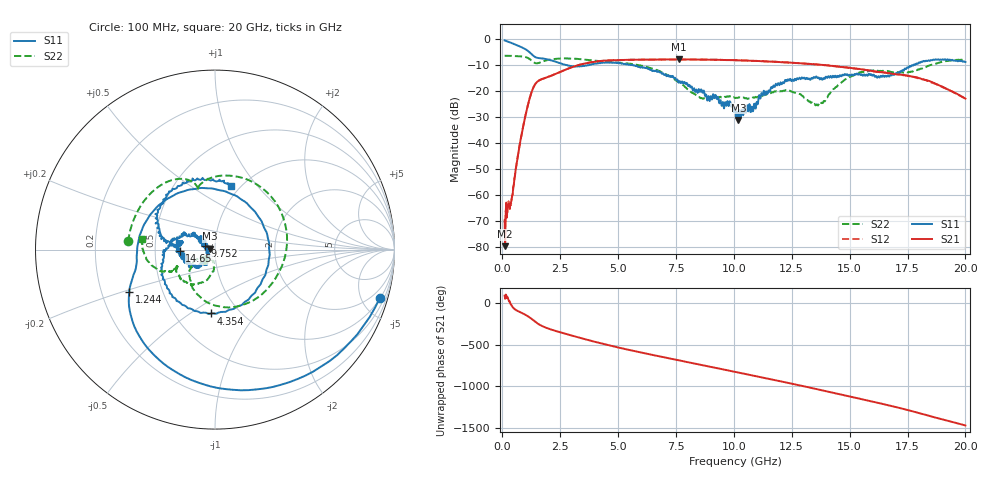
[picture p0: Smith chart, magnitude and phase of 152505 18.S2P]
!  2-Port S-parameters saved by WinCal
! VAR MeasName=S-Parameters (CALIBRATED_DATA) read from VNA (N5230C)
! VAR MeasDate=4/10/2015 9:30:06 AM
! VAR NAME=152505 18
! VAR FILENAME=152505 18.S2P
! VAR DATE=4/10/2015 9:30:06 AM
! VAR PHYS_PORTS=1,2
# Hz S DB R 50
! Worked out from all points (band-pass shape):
!   801 points, 100 MHz to 20 GHz, reference 50 ohm
!   highest |S21| = -7.69 dB at 7.637 GHz (marker M1); lowest = -79.7 dB at 124.9 MHz (marker M2)
!   |S21| within 3 dB of the highest: 3.005 GHz to 14.74 GHz (11.74 GHz wide, 132 % of centre)
!   lowest |S11| = -31.1 dB at 10.2 GHz (marker M3), VSWR 1.06, Z = 47.3 + j0.409 ohm
!   |S11| at or under -10 dB: 2.825 GHz to 3.663 GHz (838.2 MHz wide, 25.8 % of centre); 5.659293 GHz to 5.686808 GHz (27.51 MHz wide, 0.485 % of centre); 5.713 GHz to 17.68 GHz (11.97 GHz wide, 102 % of centre)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
!   |S22| runs from -25.5 to -6.3 dB; largest |S21 - S12| = 0.0066
!   S11 on the Smith chart (normalised r, x): 100 MHz: 1.05, -6.80; 1.244 GHz: 0.32, -0.21; 4.354 GHz: 0.74, -0.61; 9.752 GHz: 0.89, +0.03; 14.65 GHz: 0.67, -0.01; 20 GHz: 0.90, +0.75
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1e8  -0.38 -16.4  -69.70 88.3  -74.46 74.5  -6.29 174.6
1.24875e8  -0.46 -20.0  -79.70 51.0  -71.72 77.8  -6.28 173.3
3.985e8  -1.36 -57.5  -61.89 -25.7  -61.80 -28.8  -6.33 158.4
5.975e8  -2.07 -82.4  -49.14 -86.6  -48.94 -86.3  -6.38 147.5
1.24425e9  -5.48 -154.0  -20.85 173.4  -20.81 173.3  -7.97 108.6
2.43825e9  -9.00 107.0  -12.76 12.8  -12.75 12.5  -7.37 68.7
3.43325e9  -10.32 -10.6  -9.52 -65.3  -9.54 -65.2  -7.63 19.3
4.353625e9  -8.95 -93.9  -8.21 -132.1  -8.20 -132.2  -8.47 -20.5
5.398375e9  -9.53 -150.7  -7.86 160.0  -7.85 160.0  -9.24 -63.1
6.741625e9  -12.23 165.9  -7.76 80.6  -7.74 80.2  -12.01 -119.5
7.637125e9  -16.32 145.3  -7.69 28.9  -7.72 29.2  -16.52 -147.8
8.582375e9  -19.24 140.0  -7.77 -24.8  -7.72 -24.9  -22.62 -143.0
9.7515e9  -24.47 162.5  -7.94 -91.4  -7.94 -91.7  -22.03 -130.4
1.005e10  -26.15 178.2  -7.98 -108.9  -8.01 -109.0  -22.51 -130.6
1.019925e10  -31.07 171.1  -8.04 -117.6  -8.07 -117.3  -22.39 -130.2
1.15425e10  -20.20 -127.9  -8.52 164.9  -8.51 165.0  -20.65 -124.6
1.338325e10  -15.03 -165.8  -9.51 55.7  -9.46 55.7  -24.31 -138.4
1.465188e10  -14.16 -177.4  -10.60 -22.5  -10.56 -22.6  -16.54 -100.9
1.559712e10  -13.78 170.7  -11.60 -82.5  -11.64 -82.2  -12.52 -126.4
1.669162e10  -14.19 174.0  -12.98 -152.5  -13.03 -153.3  -12.30 -152.2
1.828362e10  -8.26 145.4  -15.62 93.0  -15.61 93.1  -10.63 -155.1
2e10  -8.69 76.1  -22.83 -34.2  -22.87 -33.3  -7.78 171.9
